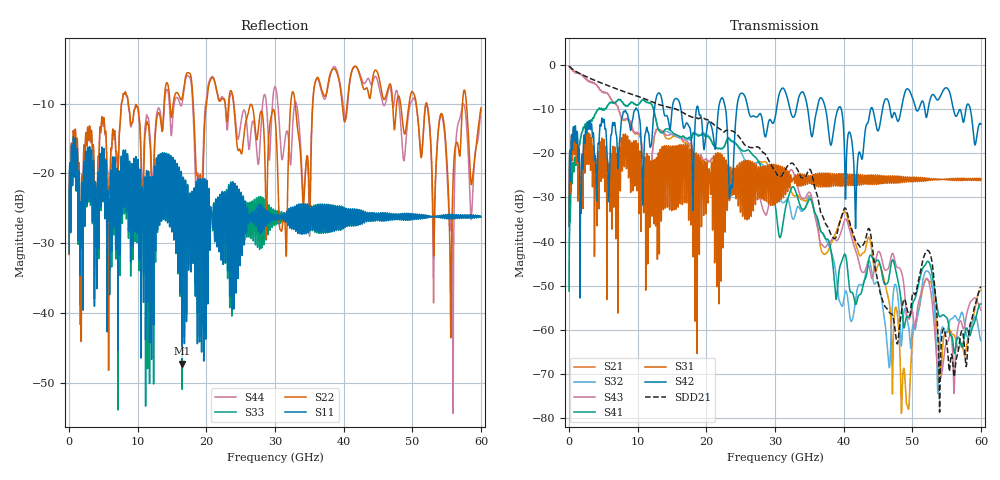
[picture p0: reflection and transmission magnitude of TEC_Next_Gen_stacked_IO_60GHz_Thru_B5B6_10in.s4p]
!! CHANNEL DESCRIPTION:  Next Generation 28Gbps Press-fit Stacked I/O Connector
!!  with 10" 5-6-5 Megtron 6 Stripline trace on host side and 1.25" 7-5-7 Megtron 6 Microstrip trace on plug side
!! HOST PCB DESCRIPTION:  PCB thickness 3.425 mm
!!  26 Layer Board, 15 GND planes, 4 Layer route-out on Layers 7,11,17,21, 8mil stub on vias
!!  Pairs on following layers
!!  Layer 07 - A02A03 A14A15 D05D06
!!  Layer 11 - D020D3 C05C06 D14D15
!!  Layer 17 - C02C03 B05B06 C14C15
!!  Layer 21 - B02B03 A05A06 B14B15
!! CONNECTOR DESCRIPTION:  Next Generation 28Gbps Press-fit Stacked I/O Connector
!! PLUG-IN CARD DESCRIPTION:  PCB thickness 1mm thick
!!  6 Layer Board, 4 GND planes, 0.35 x 1.4mm mating pads
!!  Micro-strip diff traces referenced to GND plane 3mils down, 2nd GND plane 17mils from top of board
!!  PCB GND planes are symmetric
!! MODEL DESCRIPTION: TE Connectivity S-parameter model produced from Macro-model, Extracted .s4p THRU (PAIR B05B06)
!! MODEL DATE: 5/15/2014 CR32f, FPR23
!! MODEL STATUS: Developmental
!! MODEL GEOMETRY: 4 Rows - Rows A, B, C, D. 3 pairs in each row, 12 total pairs
!! MODEL FREQUENCY RANGE: DC to 60 GHz in 10 MHz frequency steps
!! MODEL EDGE RATE LIMITATION: 8.33 ps (Using conservative 0.5/Fmax rule of thumb)
!! TIME-DOMAIN TRANSFORM CAUTIONS:
!! 1.) Do not simulate transient edge rates faster than the number listed above.  Edge
!!  rates faster than this number contain significant spectral content at frequencies
!!  above the model's highest frequency.
!! 2.) Even when simulating edge rates that are slower than the number listed above, be
!!  aware that the best time resolution possible with a direct iFFT is (1 / 2Fmax).
!!  As a result, time resolution is typically not adequate for most time-domain
!!  simulations unless tricks such as frequency-domain zero-padding and windowing are
!!  used to minimize leakage and aliasing.
!! 3.) Because the model has a uniform frequency step, a direct iFFT will result in an
!!  impulse that that has a time length given by either (1 / Fstep) or (1 / 2Fstep),
!!  depending on the transform being used.  Care has been taken in selecting the
!!  frequency step to ensure a settled impulse response for the model.  Therefore,
!!  convolution with the model's impulse response should present no issues.  However,
!!  if directly concatenating s-parameter models in the frequency domain a user must
!!  either interpolate necessary interim frequencies or complete impulse response
!!  zero-padding.  Impulse response zero-padding is more difficult, but more accurate.
!! PORT DEFINITIONS:
!! Port  1  ----->  Host B05		B05 Module <-----  Port  2
!! Port  3  ----->  Host B06		B06 Module <-----  Port  4
! Touchstone data
! Created: 29-Sep-2014 by IdEM R2011 (7.0.3)
# Hz S MA R 50
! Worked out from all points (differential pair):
!   6000 points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, 10 MHz to 60 GHz, reference 50 ohm
!   strongest paths, dB at 10 MHz, 15.01 GHz, 30.01 GHz, 45.01 GHz, 60 GHz:
!     S42: -36.6, -10.1, -12.0, -14.9, -13.4
!     S31: -36.6, -24.0, -30.4, -25.4, -25.8
!     S41: -51.2, -15.1, -31.3, -44.2, -54.1
!     S43: -0.2, -15.6, -30.7, -42.4, -55.6
!     S32: -51.2, -15.8, -28.3, -49.2, -62.5
!     S21: -0.2, -16.3, -24.3, -45.3, -51.1
!   taken as a pair (ports 3,1 in; 4,2 out), SDD21 dB: -0.2, -9.7, -24.1, -49.3, -50.2
!   lowest |S11| = -47.3 dB at 16.49 GHz (marker M1), VSWR 1.01, Z = 49.6 - j0.246 ohm
!   |S11| at or under -10 dB: start of sweep to end of sweep
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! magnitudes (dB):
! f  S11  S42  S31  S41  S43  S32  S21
! 10 MHz  -31.4  -36.6  -36.6  -51.2  -0.2  -51.2  -0.2
! 4.21 GHz  -19.9  -18.3  -19.6  -10.1  -4.9  -10.1  -4.9
! 16.49 GHz  -47.3  -12.3  -29.7  -16.1  -16.6  -16.5  -17.0
! 43.71 GHz  -26.6  -11.9  -24.9  -43.8  -45.6  -44.3  -39.0
! 49.33 GHz  -26.6  -5.4  -25.3  -57.1  -57.2  -58.2  -77.4
! 51.92 GHz  -26.1  -11.0  -26.0  -45.3  -48.9  -46.9  -48.7
! 60 GHz  -26.3  -13.4  -25.8  -54.1  -55.6  -62.5  -51.1
